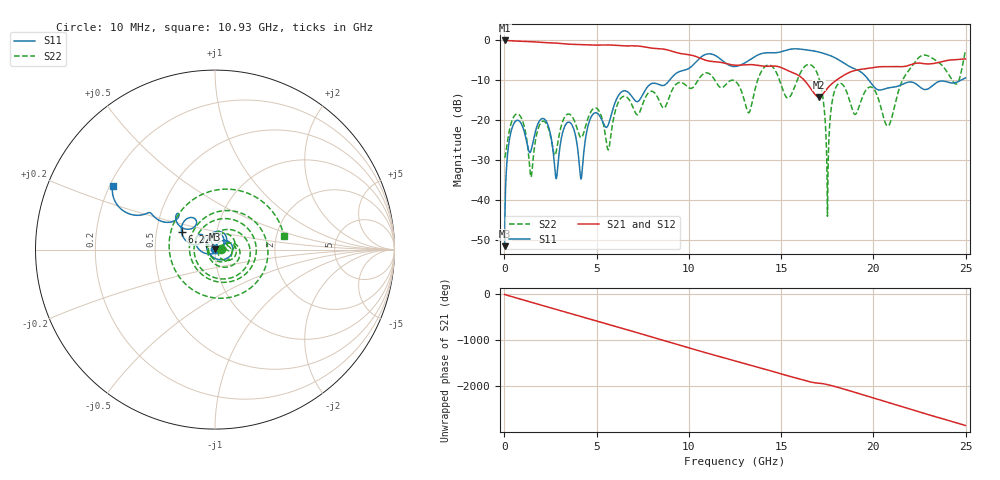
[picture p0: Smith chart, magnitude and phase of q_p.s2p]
!Keysight Technologies,N5245B,MY57181346,A.12.70.07
!Automatic Fixture Removal (AFR)
!Date: Wednesday, November 07, 2018 11:51:18 AM
!S2P File: Measurements: S11,S21,S12,S22:
# MHz S  RI  R 50
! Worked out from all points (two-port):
!   2499 points, 10 MHz to 24.99 GHz, reference 50 ohm
!   highest |S21| = 0.00 dB at 10 MHz (marker M1); lowest = -14.2 dB at 17.04 GHz (marker M2)
!   |S21| within 3 dB of the highest: start of sweep to 9.295 GHz
!   lowest |S11| = -51.7 dB at 10 MHz (marker M3), VSWR 1.01, Z = 50.1 + j0.222 ohm
!   |S11| at or under -10 dB: start of sweep to 8.948 GHz; 19.76 GHz to 24.74 GHz (4.98 GHz wide, 22.4 % of centre)
!   |S22| runs from -44.1 to -2.5 dB; largest |S21 - S12| = 1.4e-15
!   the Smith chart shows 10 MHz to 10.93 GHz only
!   S11 on the Smith chart (normalised r, x): 10 MHz: 1.00, +0.00; 6.22 GHz: 0.67, +0.14; 10.93 GHz: 0.21, +0.27
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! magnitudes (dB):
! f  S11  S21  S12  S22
! 10 MHz  -51.7  0.0  0.0  -29.5
! 230 MHz  -26.2  -0.1  -0.1  -23.5
! 640 MHz  -20.1  -0.2  -0.2  -18.5
! 1.44 GHz  -27.7  -0.3  -0.3  -34.3
! 2.17 GHz  -19.8  -0.5  -0.5  -20.4
! 2.82 GHz  -34.6  -0.7  -0.7  -27.6
! 3.53 GHz  -20.6  -0.9  -0.9  -18.5
! 4.18 GHz  -34.3  -1.0  -1.0  -24.4
! 4.73 GHz  -19.0  -1.1  -1.1  -17.6
! 5.64 GHz  -21.1  -1.1  -1.1  -27.4
! 6.22 GHz  -13.5  -1.3  -1.3  -15.1
! 8.34 GHz  -11.0  -2.1  -2.1  -14.6
! 10.93 GHz  -3.5  -5.0  -5.0  -8.1
! 12.5 GHz  -6.5  -6.2  -6.2  -10.2
! 13.24 GHz  -5.1  -6.1  -6.1  -18.2
! 16.67 GHz  -2.6  -12.5  -12.5  -6.3
! 17.04 GHz  -2.9  -14.2  -14.2  -9.3
! 17.51 GHz  -3.6  -12.0  -12.0  -44.1
! 18.14 GHz  -4.9  -9.5  -9.5  -10.8
! 20.83 GHz  -11.9  -6.6  -6.6  -21.4
! 22.45 GHz  -11.4  -5.7  -5.7  -4.3
! 24.99 GHz  -9.4  -4.6  -4.6  -2.5
